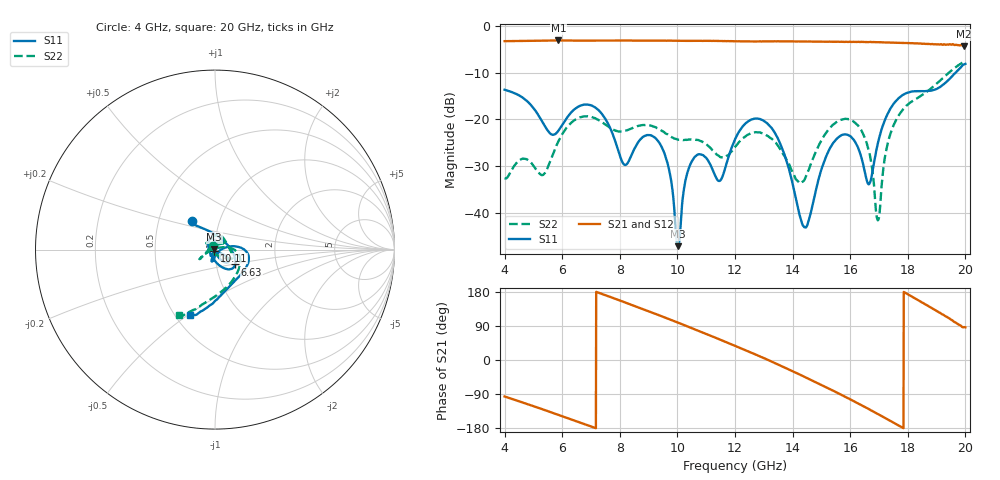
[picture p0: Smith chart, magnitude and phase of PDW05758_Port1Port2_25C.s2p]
!Agilent Technologies,E8361A,US43140610,A.07.50.67
!Agilent E8361A: A.07.50.67
!Date: Friday, February 28, 2014 12:27:08
!Correction: S11(Full 2 Port(1,2))
!S21(Full 2 Port(1,2))
!S12(Full 2 Port(1,2))
!S22(Full 2 Port(1,2))
!S2P File: Measurements: S11, S21, S12, S22:
!Power divider measured mounted on 10mil RO4350 with coaxial edge launch connectors.  Coaxial connectors have been gated out.  Unused port was externally terminated
!with coaxial termination.  Measurement reference plane placed at the part edge.  The loss of the test board and connectors has been removed.
!Port one = common port
!Port two = output port
# GHz S MA R 50
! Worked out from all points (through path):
!   1601 points, 4 GHz to 20 GHz, reference 50 ohm
!   highest |S21| = -3.15 dB at 5.87 GHz (marker M1); lowest = -4.4 dB at 19.94 GHz (marker M2)
!   lowest |S11| = -47.1 dB at 10.02 GHz (marker M3), VSWR 1.01, Z = 49.6 + j0.097 ohm
!   |S11| at or under -10 dB: start of sweep to 19.66 GHz
!   |S22| runs from -41.6 to -7.6 dB; largest |S21 - S12| = 0.032
!   S11 on the Smith chart (normalised r, x): 4 GHz: 0.73, +0.25; 6.63 GHz: 1.23, -0.21; 10.11 GHz: 0.99, -0.01; 20 GHz: 0.59, -0.51
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4  0.2069 129.1  0.6839 -96.3  0.684 -96.4  0.02343 119.0
5.87  0.07559 18.7  0.6959 -144.9  0.696 -144.9  0.0583 -45.0
6.63  0.1399 -36.4  0.6925 -165.5  0.6909 -165.4  0.1051 -29.2
6.67  0.1411 -37.9  0.6926 -166.5  0.6905 -166.5  0.1058 -28.7
8.17  0.03255 -156.9  0.6935 152.2  0.6913 152.4  0.07513 41.3
9.34  0.05793 97.4  0.6932 118.8  0.6927 118.8  0.07936 88.1
9.73  0.02712 87.3  0.6918 107.3  0.691 107.4  0.0662 105.4
10.02  0.004402 167.2  0.6906 98.6  0.69 98.8  0.06068 122.1
10.11  0.007191 -131.0  0.6903 95.9  0.6891 96.0  0.06024 127.0
10.54  0.03718 -122.7  0.6892 83.0  0.6886 83.0  0.06091 142.7
11.47  0.02194 -79.5  0.6866 54.1  0.6864 54.2  0.03978 107.0
12  0.06109 -30.1  0.6817 37.3  0.6817 37.2  0.05062 51.5
13.13  0.08977 -52.2  0.6806 0.8  0.6808 0.6  0.06647 30.7
14.36  0.007297 -92.1  0.6783 -42.4  0.6777 -42.4  0.02162 139.1
14.67  0.01137 -87.6  0.6767 -53.6  0.6754 -53.7  0.03563 -176.8
15.38  0.05401 -96.5  0.6743 -80.0  0.671 -79.8  0.08619 -149.7
16.17  0.05752 -108.7  0.6721 -110.5  0.6719 -110.2  0.09181 -150.5
16.64  0.02018 -54.1  0.6677 -129.3  0.6691 -129.2  0.04684 -159.6
16.96  0.05532 10.5  0.6667 -142.5  0.6681 -142.4  0.008332 111.4
17.34  0.1206 8.2  0.6611 -158.4  0.6624 -158.0  0.06123 13.1
19.94  0.3844 -108.5  0.6016 86.6  0.5931 84.4  0.4122 -117.5
20  0.3912 -110.5  0.6043 86.1  0.5817 84.0  0.4162 -118.7
